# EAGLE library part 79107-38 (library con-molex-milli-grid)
RECEPTACAL
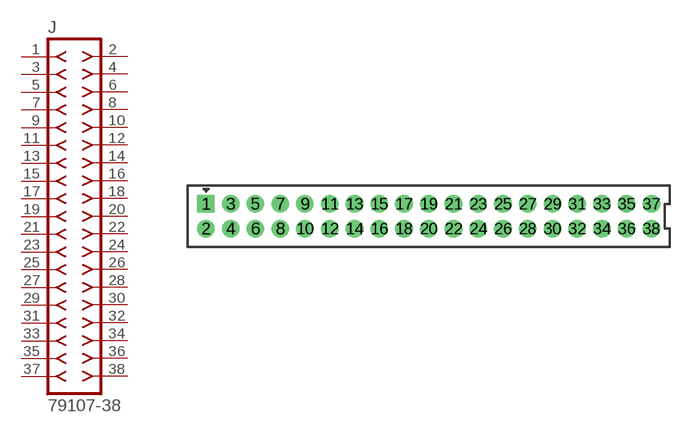
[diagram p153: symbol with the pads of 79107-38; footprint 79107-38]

Designator prefix J

## 79107-38  [79107-38]
1  1  pas
2  2  pas
3  3  pas
4  4  pas
5  5  pas
6  6  pas
7  7  pas
8  8  pas
9  9  pas
10  10  pas
11  11  pas
12  12  pas
13  13  pas
14  14  pas
15  15  pas
16  16  pas
17  17  pas
18  18  pas
19  19  pas
20  20  pas
21  21  pas
22  22  pas
23  23  pas
24  24  pas
25  25  pas
26  26  pas
27  27  pas
28  28  pas
29  29  pas
30  30  pas
31  31  pas
32  32  pas
33  33  pas
34  34  pas
35  35  pas
36  36  pas
37  37  pas
38  38  pas

## Footprint 79107-38 (pad centres in mm)
RECEPTACAL Dual Row, Vertical, Through-Hole
drill 0.914 square: 1 -18,1
drill 0.914: 2 -18,-1; 3 -16,1; 4 -16,-1; 5 -14,1; 6 -14,-1; 7 -12,1; 8 -12,-1; 9 -10,1; 10 -10,-1; 11 -8,1; 12 -8,-1; 13 -6,1; 14 -6,-1; 15 -4,1; 16 -4,-1; 17 -2,1; 18 -2,-1; 19 0,1; 20 0,-1; 21 2,1; 22 2,-1; 23 4,1; 24 4,-1; 25 6,1; 26 6,-1; 27 8,1; 28 8,-1; 29 10,1; 30 10,-1; 31 12,1; 32 12,-1; 33 14,1; 34 14,-1; 35 16,1; 36 16,-1; 37 18,1; 38 18,-1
